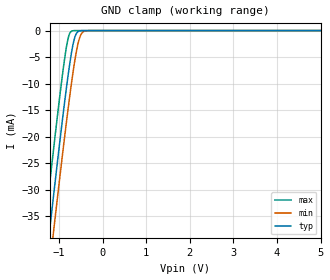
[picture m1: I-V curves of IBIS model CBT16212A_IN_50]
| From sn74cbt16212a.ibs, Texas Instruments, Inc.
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[Model]   CBT16212A_IN_50
Model_type  Input
Vinl = 0.8
Vinh = 2.0
| variable   typ   min   max
C_comp   1.52pF   1.03pF   4.40pF
[Temperature Range]   40   100   -40
| Ambient temperature   25   85   -40
[Voltage range]   5   4.5   5.5
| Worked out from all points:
|   GND clamp passes 1 mA (typ) near -0.63 V on its own axis
[GND Clamp]
| CBT16212A_IN_50
|   Voltage   I(typ)   I(min)   I(max)
-5V       -327.3mA   -333.4mA   -319.5mA
-1.365V   -48.74mA   -55.5mA    -40.02mA
-1.325V   -45.78mA   -52.55mA   -37.05mA
-1.215V   -37.7mA    -44.48mA   -28.94mA
-1.125V   -31.16mA   -37.94mA   -22.41mA
-850mV    -12.12mA   -18.65mA   -4.155mA
-780mV    -7.786mA   -14.05mA   -1.142mA
-710mV    -4.012mA   -9.712mA   -111.3uA
-625mV    -977.3uA   -5.058mA   -3.524uA
-540mV    -102.7uA   -1.712mA   -103.7nA
-380mV    -770.6nA   -48.7uA    -140.6pA
5V        35.04pA    2.714nA    24.17pA
